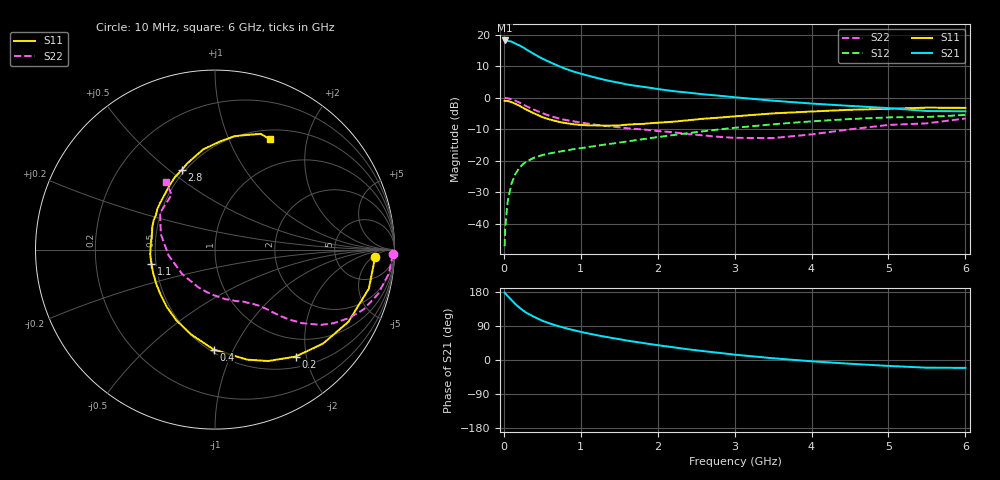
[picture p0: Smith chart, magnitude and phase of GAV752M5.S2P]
! Infineon Technologies  Discrete & RF Semiconductors
! BF775
! Si NPN RF Bipolar Junction Transistor in SOT23
! VCE = 0.75 V  IC = 2.5 mA
! Common Emitter S-Parameters:  May  1996
# GHz  S  MA  R  50
!  f  S11  S21  S12  S22
! GHz  MAG  ANG  MAG  ANG  MAG  ANG  MAG  ANG
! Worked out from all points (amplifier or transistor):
!   36 points, 10 MHz to 6 GHz, reference 50 ohm
!   highest |S21| = 18.1 dB at 10 MHz (marker M1)
!   |S21| within 3 dB of that: start of sweep to 301.8 MHz
!   unconditionally stable (mu >= 1): 956.1 MHz to end of sweep
!   at 250 MHz: K = 0.34, MSG = 18.5 dB, |S12| = -21.1 dB
!   at 1.4 GHz: K = 1.18, MAG = 7.3 dB, |S12| = -14.6 dB
!   at 6 GHz: K = 1.07, MAG = -1.0 dB, |S12| = -5.5 dB
!   S11 on the Smith chart (normalised r, x): 10 MHz: 15, -6; 200 MHz: 0.67, -1.81; 400 MHz: 0.52, -0.84; 1.1 GHz: 0.47, -0.08; 2.8 GHz: 0.48, +0.56; 6 GHz: 0.62, +1.43
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0.01  0.8904 -2.8  8.066 178.1  0.0044 87.8  0.9929 -1.5
0.02  0.8872 -5.9  7.968 175.4  0.0091 83.5  0.9864 -3.2
0.05  0.8844 -14.2  7.925 168.8  0.0225 81.9  0.9777 -7.8
0.1  0.8453 -28.4  7.736 158.1  0.0434 74.3  0.9418 -15.2
0.15  0.7978 -41.0  7.199 147.5  0.0615 66.7  0.8929 -21.9
0.2  0.7463 -53.0  6.754 138.7  0.0764 61.2  0.8383 -27.1
0.25  0.6879 -64.5  6.266 130.5  0.088 56.2  0.7779 -31.8
0.3  0.6383 -73.8  5.727 123.8  0.0977 52.8  0.724 -35.4
0.4  0.5568 -90.8  4.851 113.2  0.1124 47.4  0.6367 -40.1
0.5  0.4915 -105.7  4.153 103.6  0.1226 43.9  0.5669 -43.4
0.6  0.4489 -118.7  3.644 96.2  0.1305 42.1  0.5127 -45.7
0.7  0.4171 -130.2  3.221 89.8  0.1374 41.0  0.4735 -47.4
0.9  0.3791 -149.7  2.603 79.0  0.1518 40.0  0.4215 -50.1
1.1  0.3629 -167.6  2.222 70.0  0.1647 40.2  0.3858 -53.1
1.3  0.3587 178.2  1.929 62.0  0.1788 40.5  0.3576 -56.3
1.6  0.3722 159.7  1.62 51.3  0.2014 41.0  0.3271 -62.1
2.2  0.4142 133.1  1.268 33.7  0.2544 39.4  0.2822 -78.3
2.8  0.4811 112.5  1.072 18.8  0.3129 35.2  0.2384 -103.0
3.5  0.5618 96.8  0.894 4.6  0.3776 27.6  0.228 -143.6
4.5  0.6409 80.3  0.739 -9.9  0.4575 15.1  0.3137 164.1
5.5  0.6932 68.4  0.613 -20.3  0.4934 1.3  0.3905 128.1
6  0.6872 63.4  0.607 -20.8  0.5315 -2.5  0.4666 126.2
